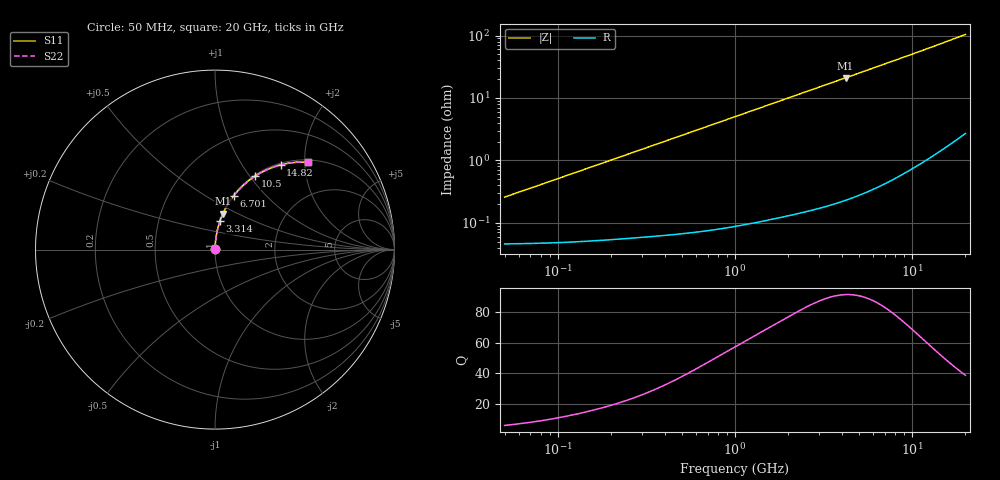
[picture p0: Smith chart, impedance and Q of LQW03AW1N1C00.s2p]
!Murata Part Number: LQW03AW1N1C00
!These Parameters are Measured in Series Mode Connection
!  o--[Z]--o
!Port1  Port2
!  o-------o
!Freq. Start=50[MHz] Stop=20[GHz], 401[Steps]
# Hz S RI R 50
!Freq.(Hz) S11(Real) S11(Imag) S21(Real) S21(Imag) S12(Real) S12(Imag) S22(Real) S22(Imag)
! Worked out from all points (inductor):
!   401 points, 50 MHz to 20 GHz, reference 50 ohm
!   read as one part in series: L = 809 pH near 51.52 MHz
!   highest Q = 91.7 at 4.212 GHz (marker M1), where L = 793 pH
!   S11 on the Smith chart (normalised r, x): 50 MHz: 1.00, +0.01; 3.314 GHz: 1.00, +0.33; 6.701 GHz: 1.01, +0.67; 10.5 GHz: 1.02, +1.06; 14.82 GHz: 1.03, +1.51; 20 GHz: 1.05, +2.08
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5e7  0.000465 0.00254  0.9995 -0.00254  0.9995 -0.00254  0.000465 0.00254
5.152053e7  0.000466 0.00262  0.9995 -0.00262  0.9995 -0.00262  0.000466 0.00262
5.721585e7  0.000469 0.00291  0.9995 -0.00291  0.9995 -0.00291  0.000469 0.00291
1.364002e8  0.000548 0.00691  0.9995 -0.00691  0.9995 -0.00691  0.000548 0.00691
3.721004e8  0.000965 0.0187  0.999 -0.0187  0.999 -0.0187  0.000965 0.0187
6.380365e8  0.00174 0.0319  0.9983 -0.0319  0.9983 -0.0319  0.00174 0.0319
1e9  0.00337 0.0498  0.9966 -0.0498  0.9966 -0.0498  0.00337 0.0498
1.714689e9  0.00843 0.0848  0.9916 -0.0848  0.9916 -0.0848  0.00843 0.0848
2.179053e9  0.013 0.1071  0.987 -0.1071  0.987 -0.1071  0.013 0.1071
2.728004e9  0.0197 0.1331  0.9803 -0.1331  0.9803 -0.1331  0.0197 0.1331
3.314454e9  0.0283 0.1602  0.9717 -0.1602  0.9717 -0.1602  0.0283 0.1602
4.212059e9  0.0442 0.2002  0.9558 -0.2002  0.9558 -0.2002  0.0442 0.2002
5.352748e9  0.0689 0.2479  0.9311 -0.2479  0.9311 -0.2479  0.0689 0.2479
6.701223e9  0.1036 0.2989  0.8964 -0.2989  0.8964 -0.2989  0.1036 0.2989
7.442007e9  0.1247 0.3243  0.8753 -0.3243  0.8753 -0.3243  0.1247 0.3243
8.907419e9  0.1697 0.3686  0.8303 -0.3686  0.8303 -0.3686  0.1697 0.3686
1.050288e10  0.2218 0.408  0.7782 -0.408  0.7782 -0.408  0.2218 0.408
1.238412e10  0.2849 0.443  0.7151 -0.443  0.7151 -0.443  0.2849 0.443
1.482269e10  0.3656 0.4719  0.6344 -0.4719  0.6344 -0.4719  0.3656 0.4719
1.721783e10  0.4403 0.4853  0.5597 -0.4853  0.5597 -0.4853  0.4403 0.4853
1.940974e10  0.5031 0.4876  0.4969 -0.4876  0.4969 -0.4876  0.5031 0.4876
2e10  0.519 0.4868  0.481 -0.4868  0.481 -0.4868  0.519 0.4868
